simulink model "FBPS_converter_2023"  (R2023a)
settings: Solver=ode23t  StartTime=0.0  StopTime=0.001  MaxStep=1e-5  RelTol=1e-5
libraries: spsDiodeLib x4, spsIGBTDiodeLib x4, spsSeriesRLCBranchLib x3, spsVoltageMeasurementLib x3, simulink x2, spsDCVoltageSourceLib x1, spsLinearTransformerLib x1, spspowerguiLib x1

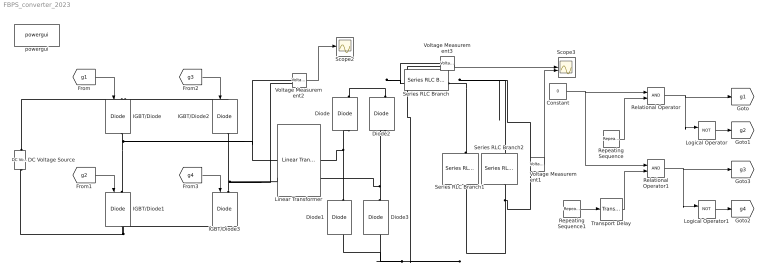
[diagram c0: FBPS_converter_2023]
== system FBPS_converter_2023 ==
  Constant : Constant  Value=0
  DC Voltage Source : spsDCVoltageSourceLib/DC Voltage Source  Amplitude=400  Measurements=None
  Diode{,1..3} (4 alike) : spsDiodeLib/Diode  Ron=0.001  Lon=0  Vf=0.8  IC=0  UseSnubber=0  Rs=500  Cs=250e-9  Measurements=on
  IGBT/Diode{,1..3} (4 alike) : spsIGBTDiodeLib/IGBT//Diode  Ron=1e-3  Rs=1e5  Cs=inf  Measurements=on
  Linear Transformer : spsLinearTransformerLib/Linear Transformer  UNITS=SI  NominalPower=[3000 50000]  winding1=[200 0.00001 0.00001]  winding2=[10 0.00001 0.00001]  ThreeWindings=off  winding3=[3.15e+05 0.7938 0.084225]  RmLm=[1000 1000]  Measurements=None  DataType=on
  Logical Operator : Logic  Operator=NOT  AllPortsSameDT=off  OutDataTypeStr=boolean
  Logical Operator1 : Logic  Operator=NOT  AllPortsSameDT=off  OutDataTypeStr=boolean
  Relational Operator : RelationalOperator  OutDataTypeStr=boolean  RndMeth=Simplest
  Relational Operator1 : RelationalOperator  OutDataTypeStr=boolean  RndMeth=Simplest
  Repeating Sequence : simulink/Sources/Repeating Sequence  rep_seq_t=[0 0.00001 0.00002]  rep_seq_y=[-400 400 -400]
  Repeating Sequence1 : simulink/Sources/Repeating Sequence  rep_seq_t=[0 0.00001 0.00002]  rep_seq_y=[-400 400 -400]
  Scope2 : Scope
  Scope3 : Scope  NumInputPorts=2
  Series RLC Branch : spsSeriesRLCBranchLib/Series RLC Branch  LConnTagsString=__new0  RConnTagsString=__new0  BranchType=L  Resistance=1  Inductance=200e-6  SetiL0=off  InitialCurrent=0  Capacitance=1e-6  Setx0=off  InitialVoltage=0  Measurements=None
  Series RLC Branch1 : spsSeriesRLCBranchLib/Series RLC Branch  LConnTagsString=__new0  RConnTagsString=__new0  BranchType=C  Resistance=1  Inductance=1e-3  SetiL0=off  InitialCurrent=0  Capacitance=47e-6  Setx0=on  InitialVoltage=12  Measurements=None
  Series RLC Branch2 : spsSeriesRLCBranchLib/Series RLC Branch  LConnTagsString=__new0  RConnTagsString=__new0  BranchType=R  Resistance=10  Inductance=1e-3  SetiL0=off  InitialCurrent=0  Capacitance=470e-6  Setx0=on  InitialVoltage=12  Measurements=None
  Transport Delay : TransportDelay  DelayTime=0.000008
  Voltage Measurement1 : spsVoltageMeasurementLib/Voltage Measurement  PhasorSimulation=off  OutputType=Complex  PSBequivalent=0
  Voltage Measurement2 : spsVoltageMeasurementLib/Voltage Measurement  PhasorSimulation=off  OutputType=Complex  PSBequivalent=0
  Voltage Measurement3 : spsVoltageMeasurementLib/Voltage Measurement  PhasorSimulation=off  OutputType=Complex  PSBequivalent=0
  powergui : spspowerguiLib/powergui  Priority=1  SimulationMode=Continuous  SampleTime=50e-6  frequency=60  Iterations=50  frequencyindice=0  Pbase=100e6  ErrMax=1e-4  UnitsV=kV  UnitsW=MW  buscounter=0  FunctionMessages=on  echomessages=on  EnableUseOfTLC=off  CurrentSourceSwitches=on  DisableSnubberDevices=on  DisableRonSwitches=on  DisableVfSwitches=on  DisplayEquations=off  AutomaticDiscreteSolvers=off  SolverType=Tustin/Backward Euler (TBE)  Interpol=off  ExternalGateDelay=off  methode=off  Ts=100  x0status=blocks  SPID=on  SwTol=0  HookPort=off  NonlinearTolerance=1e-4  nMaxIteration=100  ContinueOnMaxIteration=off  RestoreLinks=warning  ResistiveCurrentMeasurement=off  Frange=[0:2:500]  Ylog=off  Xlog=on  ShowGrid=off  save=off  variable=ZData  structure=0  ZoomFFT=off  StartTime=0.0  cycles=1  DisplayStyle=1  fundamental=60  FreqAxis=off  MaxFrequency=1000  frequencyindicesteady=1  RmsSteady=1  display=off
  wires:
  [g4] -> IGBT/Diode3/1
  [g2] -> IGBT/Diode1/1
  [g1] -> IGBT/Diode/1
  [g3] -> IGBT/Diode2/1
  Repeating Sequence/1 -> Relational Operator/2
  Constant/1 -> Relational Operator1/1, Relational Operator/1
  Relational Operator/1 -> Logical Operator/1, [g1]
  Logical Operator/1 -> [g2]
  Repeating Sequence1/1 -> Transport Delay/1
  Relational Operator1/1 -> Logical Operator1/1, [g3]
  Logical Operator1/1 -> [g4]
  Transport Delay/1 -> Relational Operator1/2
  Voltage Measurement2/1 -> Scope2/1
  Voltage Measurement3/1 -> Scope3/1
  Voltage Measurement1/1 -> Scope3/2
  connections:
  IGBT/Diode1/LConn1 -- Voltage Measurement2/LConn1 -- Linear Transformer/LConn1 -- IGBT/Diode/RConn1
  DC Voltage Source/RConn1 -- IGBT/Diode2/LConn1 -- IGBT/Diode/LConn1
  IGBT/Diode1/RConn1 -- DC Voltage Source/LConn1 -- IGBT/Diode3/RConn1
  IGBT/Diode3/LConn1 -- Voltage Measurement2/LConn2 -- Linear Transformer/LConn2 -- IGBT/Diode2/RConn1
  Series RLC Branch1/LConn1 -- Series RLC Branch2/LConn1 -- Voltage Measurement1/LConn1 -- Series RLC Branch/RConn1
  Series RLC Branch2/RConn1 -- Voltage Measurement3/LConn2 -- Diode1/LConn1 -- Diode3/LConn1 -- Series RLC Branch1/RConn1 -- Voltage Measurement1/LConn2
  Diode/RConn1 -- Voltage Measurement3/LConn1 -- Series RLC Branch/LConn1 -- Diode2/RConn1
  Diode1/RConn1 -- Linear Transformer/RConn1 -- Diode/LConn1
  Diode3/RConn1 -- Linear Transformer/RConn2 -- Diode2/LConn1
